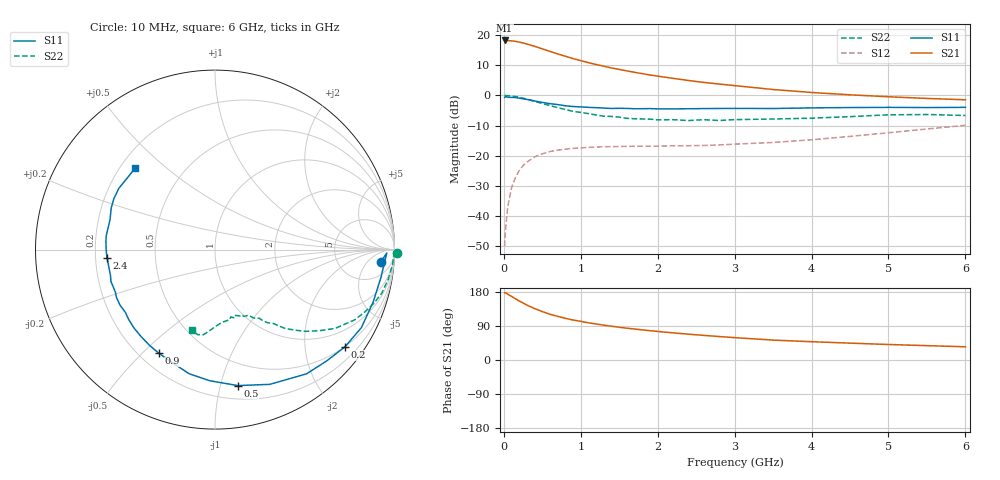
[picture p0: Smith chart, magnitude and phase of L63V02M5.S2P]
!  INFINEON TECHNOLOGIES Small Signal Semiconductors
! BFR380L3 , Si-NPN RF-Transistor in TSLP-3-1
!  Vce=3 V,  Ic=2.5 mA
! Common Emitter S-Parameters:  07. March 2005
#  GHz  S  MA  R  50
! f  S11  S21  S12  S22
! GHz  Mag  Ang  Mag  Ang  Mag  Ang  Mag  Ang
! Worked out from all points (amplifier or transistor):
!   36 points, 10 MHz to 6 GHz, reference 50 ohm
!   highest |S21| = 18.2 dB at 10 MHz (marker M1)
!   |S21| within 3 dB of that: start of sweep to 526 MHz
!   unconditionally stable (mu >= 1): 2.707 GHz to 4.652 GHz
!   at 250 MHz: K = 0.10, MSG = 20.3 dB, |S12| = -23.2 dB
!   at 1.4 GHz: K = 0.60, MSG = 13.0 dB, |S12| = -17.0 dB
!   at 6 GHz: K = 0.90, MSG = 4.2 dB, |S12| = -9.9 dB
!   S11 on the Smith chart (normalised r, x): 10 MHz: 14, -13; 200 MHz: 0.49, -2.93; 500 MHz: 0.31, -1.13; 900 MHz: 0.28, -0.56; 2.4 GHz: 0.25, -0.04; 6 GHz: 0.26, +0.40
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0.01  0.9264 -4.2  8.142 177.1  0.0032 87.2  1.015 -1.0
0.02  0.9575 -1.1  8.093 177.9  0.0057 91.1  0.9956 -2.1
0.05  0.9374 -9.6  8.119 173.8  0.0142 84.7  0.9928 -4.9
0.1  0.9284 -18.4  8.002 167.9  0.0297 81.6  0.9787 -9.8
0.15  0.9242 -28.1  7.881 161.7  0.0435 74.9  0.9605 -14.6
0.2  0.9041 -36.8  7.645 155.7  0.057 70.5  0.9344 -18.7
0.3  0.8598 -53.6  7.094 144.9  0.0788 62.3  0.8712 -26.7
0.4  0.8104 -67.9  6.519 135.6  0.0962 54.8  0.8002 -33.3
0.5  0.7681 -80.5  5.914 127.8  0.1083 49.4  0.7358 -37.9
0.6  0.7312 -92.3  5.357 120.7  0.1181 45.0  0.6794 -42.1
0.7  0.7066 -101.7  4.87 115.2  0.1244 41.8  0.6296 -45.4
0.8  0.675 -110.2  4.454 109.9  0.1292 39.0  0.5851 -48.5
0.9  0.6565 -118.5  4.081 105.5  0.1329 36.9  0.546 -50.5
1.1  0.636 -130.4  3.496 98.1  0.1382 34.2  0.501 -54.4
1.3  0.6186 -141.1  3.057 91.9  0.142 32.8  0.4541 -57.2
1.6  0.6103 -154.0  2.549 83.9  0.1437 32.2  0.4185 -62.2
2.2  0.5995 -170.9  1.921 71.6  0.1466 35.6  0.3973 -68.9
2.4  0.603 -175.7  1.77 68.2  0.1473 37.5  0.3843 -72.4
3.5  0.6083 164.0  1.255 52.5  0.1667 49.9  0.4071 -84.1
4.5  0.6309 153.3  1.025 44.5  0.2102 60.6  0.4462 -92.8
5.5  0.6308 141.3  0.893 37.9  0.2787 64.9  0.4837 -101.6
6  0.6356 134.5  0.848 34.9  0.3207 64.7  0.4661 -106.2
